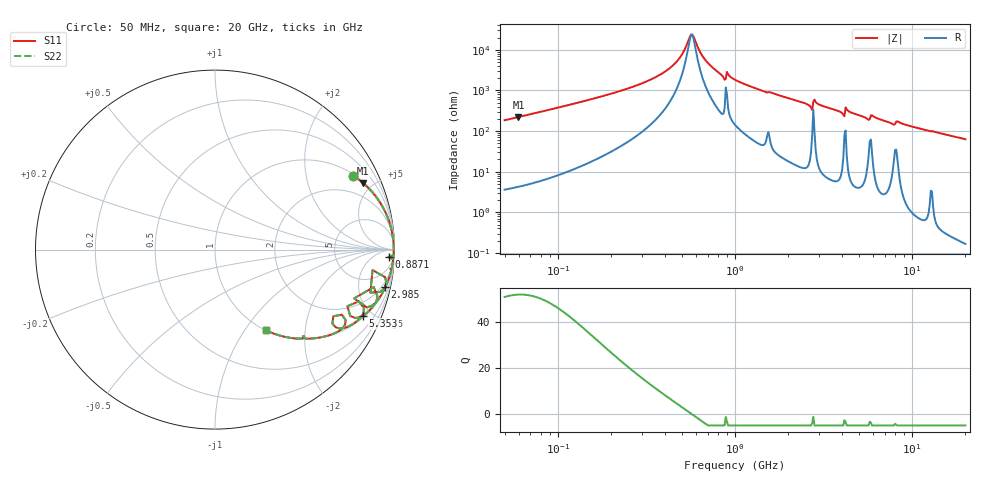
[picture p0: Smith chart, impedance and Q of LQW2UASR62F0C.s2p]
!Murata Part Number: LQW2UASR62F0C
!These Parameters are Measured in Series Mode Connection
!  o--[Z]--o
!Port1  Port2
!  o-------o
!Freq. Start=50[MHz] Stop=20[GHz], 401[Steps]
# Hz S RI R 50
!Freq.(Hz) S11(Real) S11(Imag) S21(Real) S21(Imag) S12(Real) S12(Imag) S22(Real) S22(Imag)
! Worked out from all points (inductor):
!   401 points, 50 MHz to 20 GHz, reference 50 ohm
!   read as one part in series: L = 581 nH near 51.52 MHz
!   highest Q = 52.1 at 59.85 MHz (marker M1), where L = 587 nH
!   self-resonance near 566 MHz
!   S11 on the Smith chart (normalised r, x): 50 MHz: 1.07, +3.68; 887.1 MHz: 25, -30; 2.985 GHz: 1.24, -8.97; 5.353 GHz: 1.11, -4.42; 20 GHz: 1.00, -1.26
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5e7  0.7675 0.4127  0.2325 -0.4127  0.2325 -0.4127  0.7675 0.4127
5.984554e7  0.8252 0.3703  0.1748 -0.3703  0.1748 -0.3703  0.8252 0.3703
1.364002e8  0.9609 0.1812  0.0391 -0.1812  0.0391 -0.1812  0.9609 0.1812
2.520729e8  0.9882 0.0862  0.0118 -0.0862  0.0118 -0.0862  0.9882 0.0862
3.721004e8  0.994 0.042  0.00596 -0.042  0.00596 -0.042  0.994 0.042
4.728708e8  0.9955 0.018  0.00447 -0.018  0.00447 -0.018  0.9955 0.018
5.659842e8  0.9959 0.000662  0.00413 -0.000662  0.00413 -0.000662  0.9959 0.000662
5.831961e8  0.9959 -0.00222  0.00414 0.00222  0.00414 0.00222  0.9959 -0.00222
6.380365e8  0.9957 -0.0109  0.00425 0.0109  0.00425 0.0109  0.9957 -0.0109
6.980337e8  0.9955 -0.0198  0.00454 0.0198  0.00454 0.0198  0.9955 -0.0198
8.608917e8  0.9917 -0.0467  0.00829 0.0467  0.00829 0.0467  0.9917 -0.0467
8.870719e8  0.9676 -0.0386  0.0324 0.0386  0.0324 0.0386  0.9676 -0.0386
9.278425e8  0.9932 -0.0428  0.00682 0.0428  0.00682 0.0428  0.9932 -0.0428
1e9  0.9928 -0.0539  0.00717 0.0539  0.00717 0.0539  0.9928 -0.0539
2.647493e9  0.9356 -0.2237  0.0644 0.2237  0.0644 0.2237  0.9356 -0.2237
2.728004e9  0.8656 -0.2396  0.1344 0.2396  0.1344 0.2396  0.8656 -0.2396
2.853386e9  0.9533 -0.1801  0.0467 0.1801  0.0467 0.1801  0.9533 -0.1801
2.98453e9  0.9475 -0.2099  0.0525 0.2099  0.0525 0.2099  0.9475 -0.2099
5.352748e9  0.8243 -0.3686  0.1757 0.3686  0.1757 0.3686  0.8243 -0.3686
6.034176e9  0.8281 -0.3492  0.1719 0.3492  0.1719 0.3492  0.8281 -0.3492
7.442007e9  0.7193 -0.4368  0.2807 0.4368  0.2807 0.4368  0.7193 -0.4368
2e10  0.2846 -0.4499  0.7154 0.4499  0.7154 0.4499  0.2846 -0.4499
